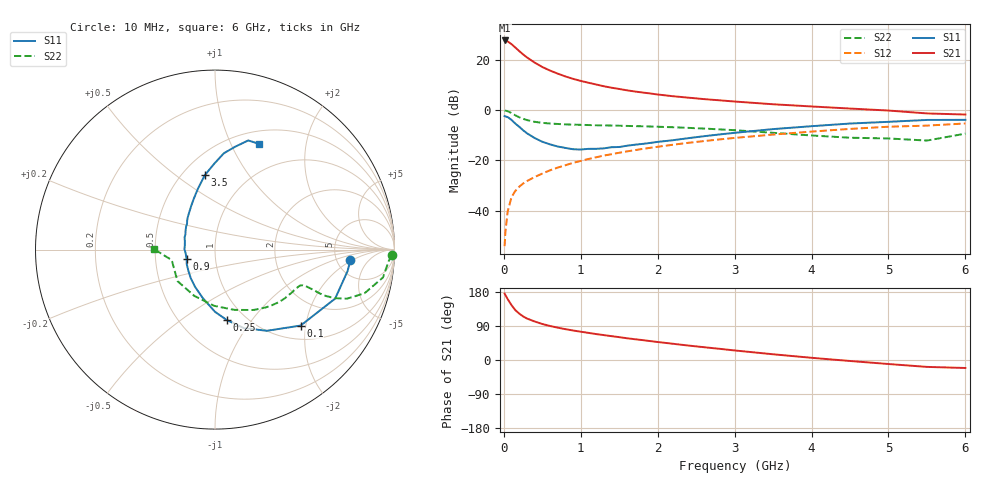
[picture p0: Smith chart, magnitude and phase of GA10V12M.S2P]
! Infineon Technologies  Discrete & RF Semiconductors
! BF775
! Si NPN RF Bipolar Junction Transistor in SOT23
! VCE = 10 V  IC = 12 mA
! Common Emitter S-Parameters:  May  1996
# GHz  S  MA  R  50
!  f  S11  S21  S12  S22
! GHz  MAG  ANG  MAG  ANG  MAG  ANG  MAG  ANG
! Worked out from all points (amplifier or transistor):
!   36 points, 10 MHz to 6 GHz, reference 50 ohm
!   highest |S21| = 27.6 dB at 10 MHz (marker M1)
!   |S21| within 3 dB of that: start of sweep to 156.5 MHz
!   unconditionally stable (mu >= 1): 601.8 MHz to 2.724 GHz
!   at 250 MHz: K = 0.69, MSG = 25.6 dB, |S12| = -29.2 dB
!   at 1.4 GHz: K = 1.09, MAG = 11.4 dB, |S12| = -17.5 dB
!   at 6 GHz: K = 0.88, MSG = 1.8 dB, |S12| = -5.3 dB
!   S11 on the Smith chart (normalised r, x): 10 MHz: 6.68, -1.85; 100 MHz: 1.31, -1.87; 250 MHz: 0.82, -0.76; 900 MHz: 0.72, -0.08; 3.5 GHz: 0.64, +0.64; 6 GHz: 0.64, +1.28
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0.01  0.7564 -4.5  23.92 175.3  0.002 80.7  0.9854 -1.8
0.02  0.7483 -9.2  23.86 171.3  0.0038 87.2  0.9693 -3.9
0.05  0.7229 -22.2  22.89 160.6  0.0098 79.1  0.9488 -9.4
0.1  0.6376 -41.6  20.18 144.7  0.0188 71.7  0.8676 -16.3
0.15  0.5369 -57.4  17.28 131.4  0.025 66.9  0.7845 -20.4
0.2  0.4661 -69.8  14.74 122.5  0.0302 64.8  0.7191 -22.1
0.25  0.3972 -80.6  12.66 115.1  0.0348 64.0  0.6693 -22.7
0.3  0.3465 -90.0  11.05 109.5  0.039 64.5  0.6318 -22.7
0.4  0.2787 -104.1  8.718 101.7  0.0469 65.6  0.5842 -22.2
0.5  0.2348 -118.4  7.118 95.0  0.055 65.8  0.5565 -22.0
0.6  0.2086 -130.4  6.059 89.8  0.0638 66.3  0.5402 -21.9
0.7  0.189 -141.9  5.266 85.4  0.0722 67.2  0.5288 -22.1
0.8  0.1772 -152.6  4.628 81.4  0.0804 67.3  0.5195 -22.5
0.9  0.167 -161.2  4.147 77.9  0.0897 67.1  0.513 -23.1
1.1  0.1699 179.5  3.469 71.6  0.107 66.8  0.5035 -25.1
1.3  0.1737 165.1  2.959 65.7  0.1249 65.8  0.4952 -27.3
1.6  0.196 146.6  2.457 57.4  0.1511 64.0  0.4836 -31.2
2.2  0.2521 124.8  1.875 42.8  0.2052 59.4  0.4554 -40.8
3.5  0.4184 97.8  1.3 15.1  0.3261 46.1  0.3532 -72.0
4.5  0.5395 84.7  1.069 -2.6  0.422 34.0  0.2823 -114.2
5.5  0.6355 73.1  0.856 -18.2  0.4907 18.9  0.2481 -166.4
6  0.6383 67.6  0.813 -21.1  0.5412 14.7  0.3401 179.5
